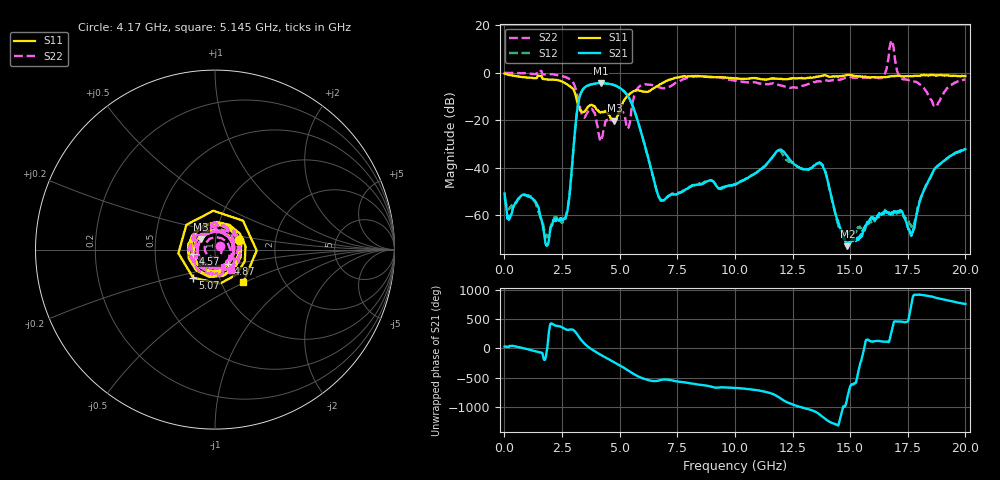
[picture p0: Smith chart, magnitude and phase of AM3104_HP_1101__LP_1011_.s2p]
!Created with skrf (http://scikit-rf.org).
# Hz S RI R 50.0
!freq ReS11 ImS11 ReS21 ImS21 ReS12 ImS12 ReS22 ImS22
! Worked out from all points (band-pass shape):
!   1601 points, 10 MHz to 20 GHz, reference 50 ohm
!   highest |S21| = -4.31 dB at 4.183 GHz (marker M1); lowest = -73.1 dB at 14.88 GHz (marker M2)
!   |S21| within 3 dB of the highest: 3.387 GHz to 5.133 GHz (1.746 GHz wide, 41 % of centre)
!   lowest |S11| = -20.2 dB at 4.77 GHz (marker M3), VSWR 1.22, Z = 42.6 + j5.11 ohm
!   |S11| at or under -10 dB: 3.105 GHz to 5.316 GHz (2.211 GHz wide, 52.5 % of centre)
!   |S22| runs from -28.9 to 13.6 dB; largest |S21 - S12| = 0.052
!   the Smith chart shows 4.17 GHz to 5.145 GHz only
!   S11 on the Smith chart (normalised r, x): 4.17 GHz: 1.30, +0.14; 4.57 GHz: 0.78, -0.04; 4.87 GHz: 1.15, -0.19; 5.07 GHz: 0.75, -0.24; 5.145 GHz: 1.27, -0.49
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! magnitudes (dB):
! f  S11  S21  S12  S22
! 10 MHz  -0.4  -50.9  -52.6  0.0
! 1.284 GHz  -2.2  -53.6  -54.0  -0.6
! 1.847 GHz  -2.9  -72.7  -68.3  -0.6
! 2.571 GHz  -4.0  -61.8  -63.2  -1.6
! 3.346 GHz  -16.3  -8.0  -8.1  -17.0
! 4.17 GHz  -16.8  -4.3  -4.4  -28.9
! 4.183 GHz  -16.8  -4.3  -4.4  -28.9
! 4.57 GHz  -18.2  -4.7  -4.8  -19.3
! 4.77 GHz  -20.2  -5.2  -5.3  -20.2
! 4.87 GHz  -19.1  -5.6  -5.7  -19.0
! 5.07 GHz  -14.0  -6.8  -6.8  -16.4
! 5.145 GHz  -12.4  -7.4  -7.4  -16.7
! 6.682 GHz  -5.3  -51.9  -52.1  -6.0
! 10.01 GHz  -2.5  -47.3  -47.2  -3.4
! 11.93 GHz  -2.5  -32.5  -32.7  -5.2
! 13.34 GHz  -2.1  -40.0  -40.0  -4.3
! 13.84 GHz  -1.2  -40.1  -39.6  -3.4
! 14.88 GHz  -0.9  -73.1  -67.5  -2.0
! 16.68 GHz  -1.6  -59.4  -58.8  7.2
! 17.69 GHz  -1.5  -67.7  -65.0  -3.6
! 18.64 GHz  -1.1  -40.9  -41.1  -13.8
! 20 GHz  -1.4  -32.3  -31.9  -2.8
